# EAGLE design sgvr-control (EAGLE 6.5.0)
CNAME: SGVR Control Board; CREVISION: 1; DESIGNER: Rian Wardana

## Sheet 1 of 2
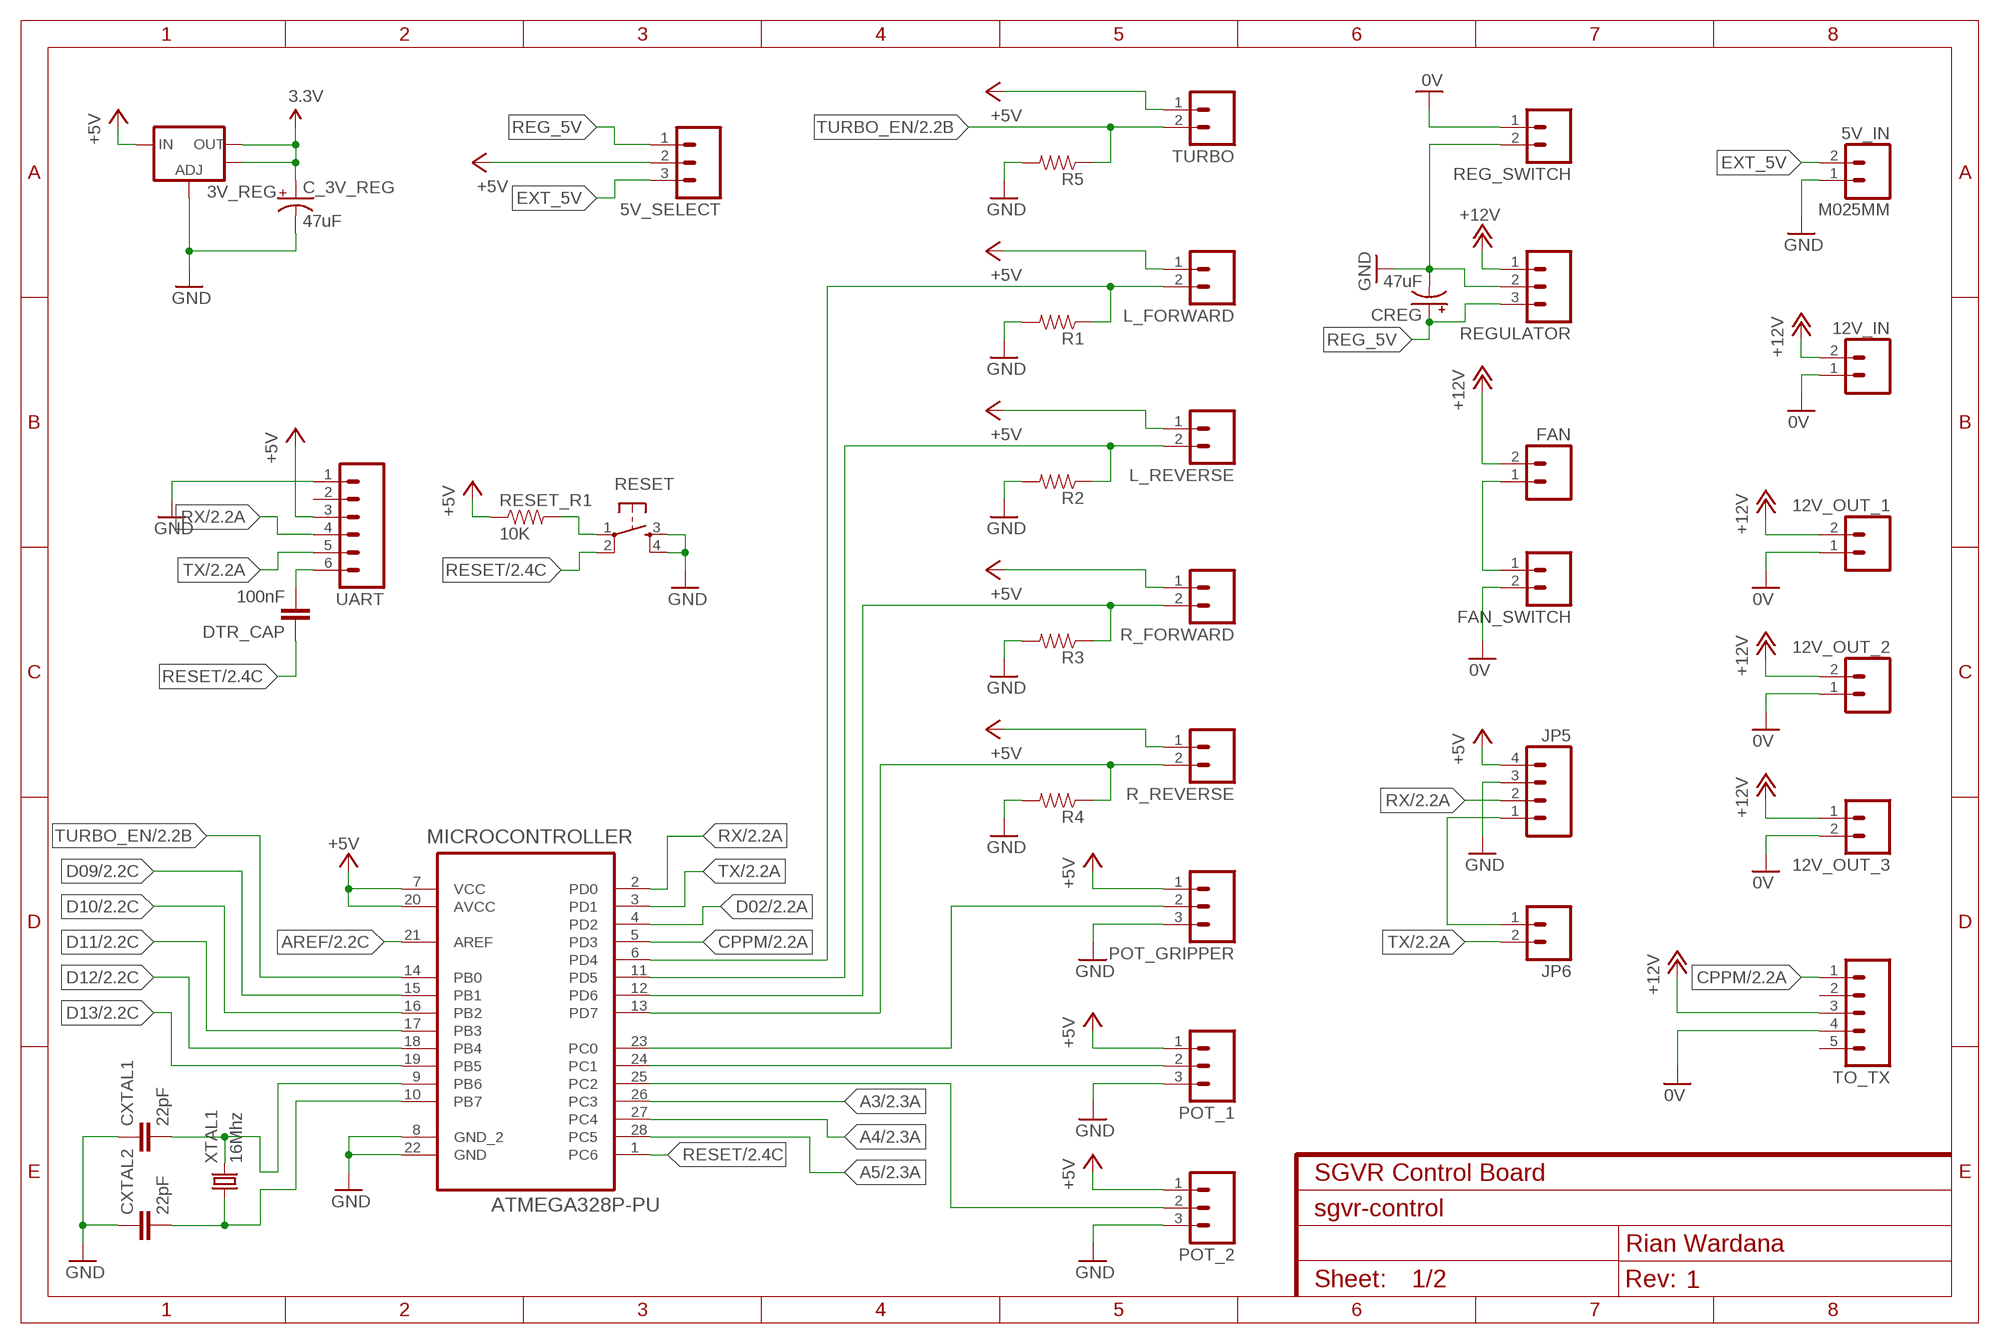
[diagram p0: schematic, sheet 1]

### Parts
3V_REG  V_REG_LM1117SOT223  [SOT223]
5V_IN  M025MM  [SCREWTERMINAL-5MM-2]
5V_SELECT  M03LOCK_LONGPADS  [1X03_LOCK_LONGPADS]
12V_IN  M025MM  [SCREWTERMINAL-5MM-2]
12V_OUT_1  M025MM  [SCREWTERMINAL-5MM-2]
12V_OUT_2  M025MM  [SCREWTERMINAL-5MM-2]
12V_OUT_3  M02LOCK_LONGPADS  [1X02_LOCK_LONGPADS]
C_3V_REG  47uF  CAP_POLPTH1  [CPOL-RADIAL-100UF-25V]
CREG  47uF  CAP_POLPTH1  [CPOL-RADIAL-100UF-25V]
CXTAL1  22pF  CAPPTH  [CAP-PTH-SMALL]
CXTAL2  22pF  CAPPTH  [CAP-PTH-SMALL]
DTR_CAP  100nF  CAPPTH  [CAP-PTH-SMALL]
FAN  M02LOCK_LONGPADS  [1X02_LOCK_LONGPADS]
FAN_SWITCH  M02LOCK_LONGPADS  [1X02_LOCK_LONGPADS]
JP5  M04LOCK_LONGPADS  [1X04_LOCK_LONGPADS]
JP6  M02LOCK_LONGPADS  [1X02_LOCK_LONGPADS]
L_FORWARD  M02LOCK_LONGPADS  [1X02_LOCK_LONGPADS]
L_REVERSE  M02LOCK_LONGPADS  [1X02_LOCK_LONGPADS]
MICROCONTROLLER  ATMEGA328P-PU  [DIP254P762X457-28]
POT_1  M03LOCK_LONGPADS  [1X03_LOCK_LONGPADS]
POT_2  M03LOCK_LONGPADS  [1X03_LOCK_LONGPADS]
POT_GRIPPER  M03LOCK_LONGPADS  [1X03_LOCK_LONGPADS]
R1  RESISTORAXIAL-0.3  [AXIAL-0.3]
R2  RESISTORAXIAL-0.3  [AXIAL-0.3]
R3  RESISTORAXIAL-0.3  [AXIAL-0.3]
R4  RESISTORAXIAL-0.3  [AXIAL-0.3]
R5  RESISTORAXIAL-0.3  [AXIAL-0.3]
R_FORWARD  M02LOCK_LONGPADS  [1X02_LOCK_LONGPADS]
R_REVERSE  M02LOCK_LONGPADS  [1X02_LOCK_LONGPADS]
REG_SWITCH  M02LOCK_LONGPADS  [1X02_LOCK_LONGPADS]
REGULATOR  M03LOCK_LONGPADS  [1X03_LOCK_LONGPADS]
RESET  TAC_SWITCHPTH  [TACTILE-PTH]
RESET_R1  10K  RESISTORAXIAL-0.3  [AXIAL-0.3]
TO_TX  M05LOCK_LONGPADS  [1X05_LOCK_LONGPADS]
TURBO  M02LOCK_LONGPADS  [1X02_LOCK_LONGPADS]
UART  M06LOCK_LONGPADS  [1X06_LOCK_LONGPADS]
XTAL1  16Mhz  CRYSTALHC49UV  [HC49U-V]

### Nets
3.3V: 3V_REG.2(OUT) 3V_REG.4(OUT) C_3V_REG.1(+) ; also sheet 2
+5V: 3V_REG.3(IN) 5V_SELECT.2 JP5.4 L_FORWARD.1 L_REVERSE.1 MICROCONTROLLER.7(VCC) MICROCONTROLLER.20(AVCC) POT_1.1 POT_2.1 POT_GRIPPER.1 R_FORWARD.1 R_REVERSE.1 RESET_R1.P$1 TURBO.1 UART.3 ; also sheet 2
+12V: 12V_IN.2 12V_OUT_1.2 12V_OUT_2.2 12V_OUT_3.1 FAN.2 REGULATOR.1 TO_TX.3
A0: MICROCONTROLLER.23(PC0) POT_GRIPPER.2 ; also sheet 2
A1: MICROCONTROLLER.24(PC1) POT_1.2 ; also sheet 2
A2: MICROCONTROLLER.25(PC2) POT_2.2 ; also sheet 2
A3: MICROCONTROLLER.26(PC3) ; also sheet 2
A4: MICROCONTROLLER.27(PC4) ; also sheet 2
A5: MICROCONTROLLER.28(PC5) ; also sheet 2
AREF: MICROCONTROLLER.21(AREF) ; also sheet 2
CPPM: MICROCONTROLLER.5(PD3) TO_TX.1 ; also sheet 2
D02: MICROCONTROLLER.4(PD2) ; also sheet 2
D04: L_FORWARD.2 MICROCONTROLLER.6(PD4) R1.P$1 ; also sheet 2
D05: L_REVERSE.2 MICROCONTROLLER.11(PD5) R2.P$1 ; also sheet 2
D06: MICROCONTROLLER.12(PD6) R3.P$1 R_FORWARD.2 ; also sheet 2
D07: MICROCONTROLLER.13(PD7) R4.P$1 R_REVERSE.2 ; also sheet 2
D09: MICROCONTROLLER.15(PB1) ; also sheet 2
D10: MICROCONTROLLER.16(PB2) ; also sheet 2
D12: MICROCONTROLLER.18(PB4) ; also sheet 2
D13: MICROCONTROLLER.19(PB5) ; also sheet 2
DTR: DTR_CAP.2 UART.6
EXT_5V: 5V_IN.2 5V_SELECT.3
GND: 3V_REG.1(ADJ) 5V_IN.1 C_3V_REG.2(-) CREG.2(-) CXTAL1.1 CXTAL2.1 JP5.3 MICROCONTROLLER.8(GND_2) MICROCONTROLLER.22(GND) POT_1.3 POT_2.3 POT_GRIPPER.3 R1.P$2 R2.P$2 R3.P$2 R4.P$2 R5.P$2 REG_SWITCH.2 REGULATOR.2 RESET.3 RESET.4 UART.1 ; also sheet 2
GROUND12: 12V_IN.1 12V_OUT_1.1 12V_OUT_2.1 12V_OUT_3.2 FAN_SWITCH.2 REG_SWITCH.1 TO_TX.4 ; supply symbol labelled 0V
N$1: FAN.1 FAN_SWITCH.1
N$2: JP5.1 JP6.1
N$3: CXTAL1.2 MICROCONTROLLER.9(PB6) XTAL1.2
N$4: CXTAL2.2 MICROCONTROLLER.10(PB7) XTAL1.1
N$13: RESET.1 RESET_R1.P$2
REG_5V: 5V_SELECT.1 CREG.1(+) REGULATOR.3
RESET: DTR_CAP.1 MICROCONTROLLER.1(PC6) RESET.2 ; also sheet 2
RX: JP5.2 MICROCONTROLLER.2(PD0) UART.4 ; also sheet 2
TURBO_EN: MICROCONTROLLER.14(PB0) R5.P$1 TURBO.2 ; also sheet 2
TX: JP6.2 MICROCONTROLLER.3(PD1) UART.5 ; also sheet 2
Unconnected: MICROCONTROLLER.17(PB3) TO_TX.2 TO_TX.5 UART.2

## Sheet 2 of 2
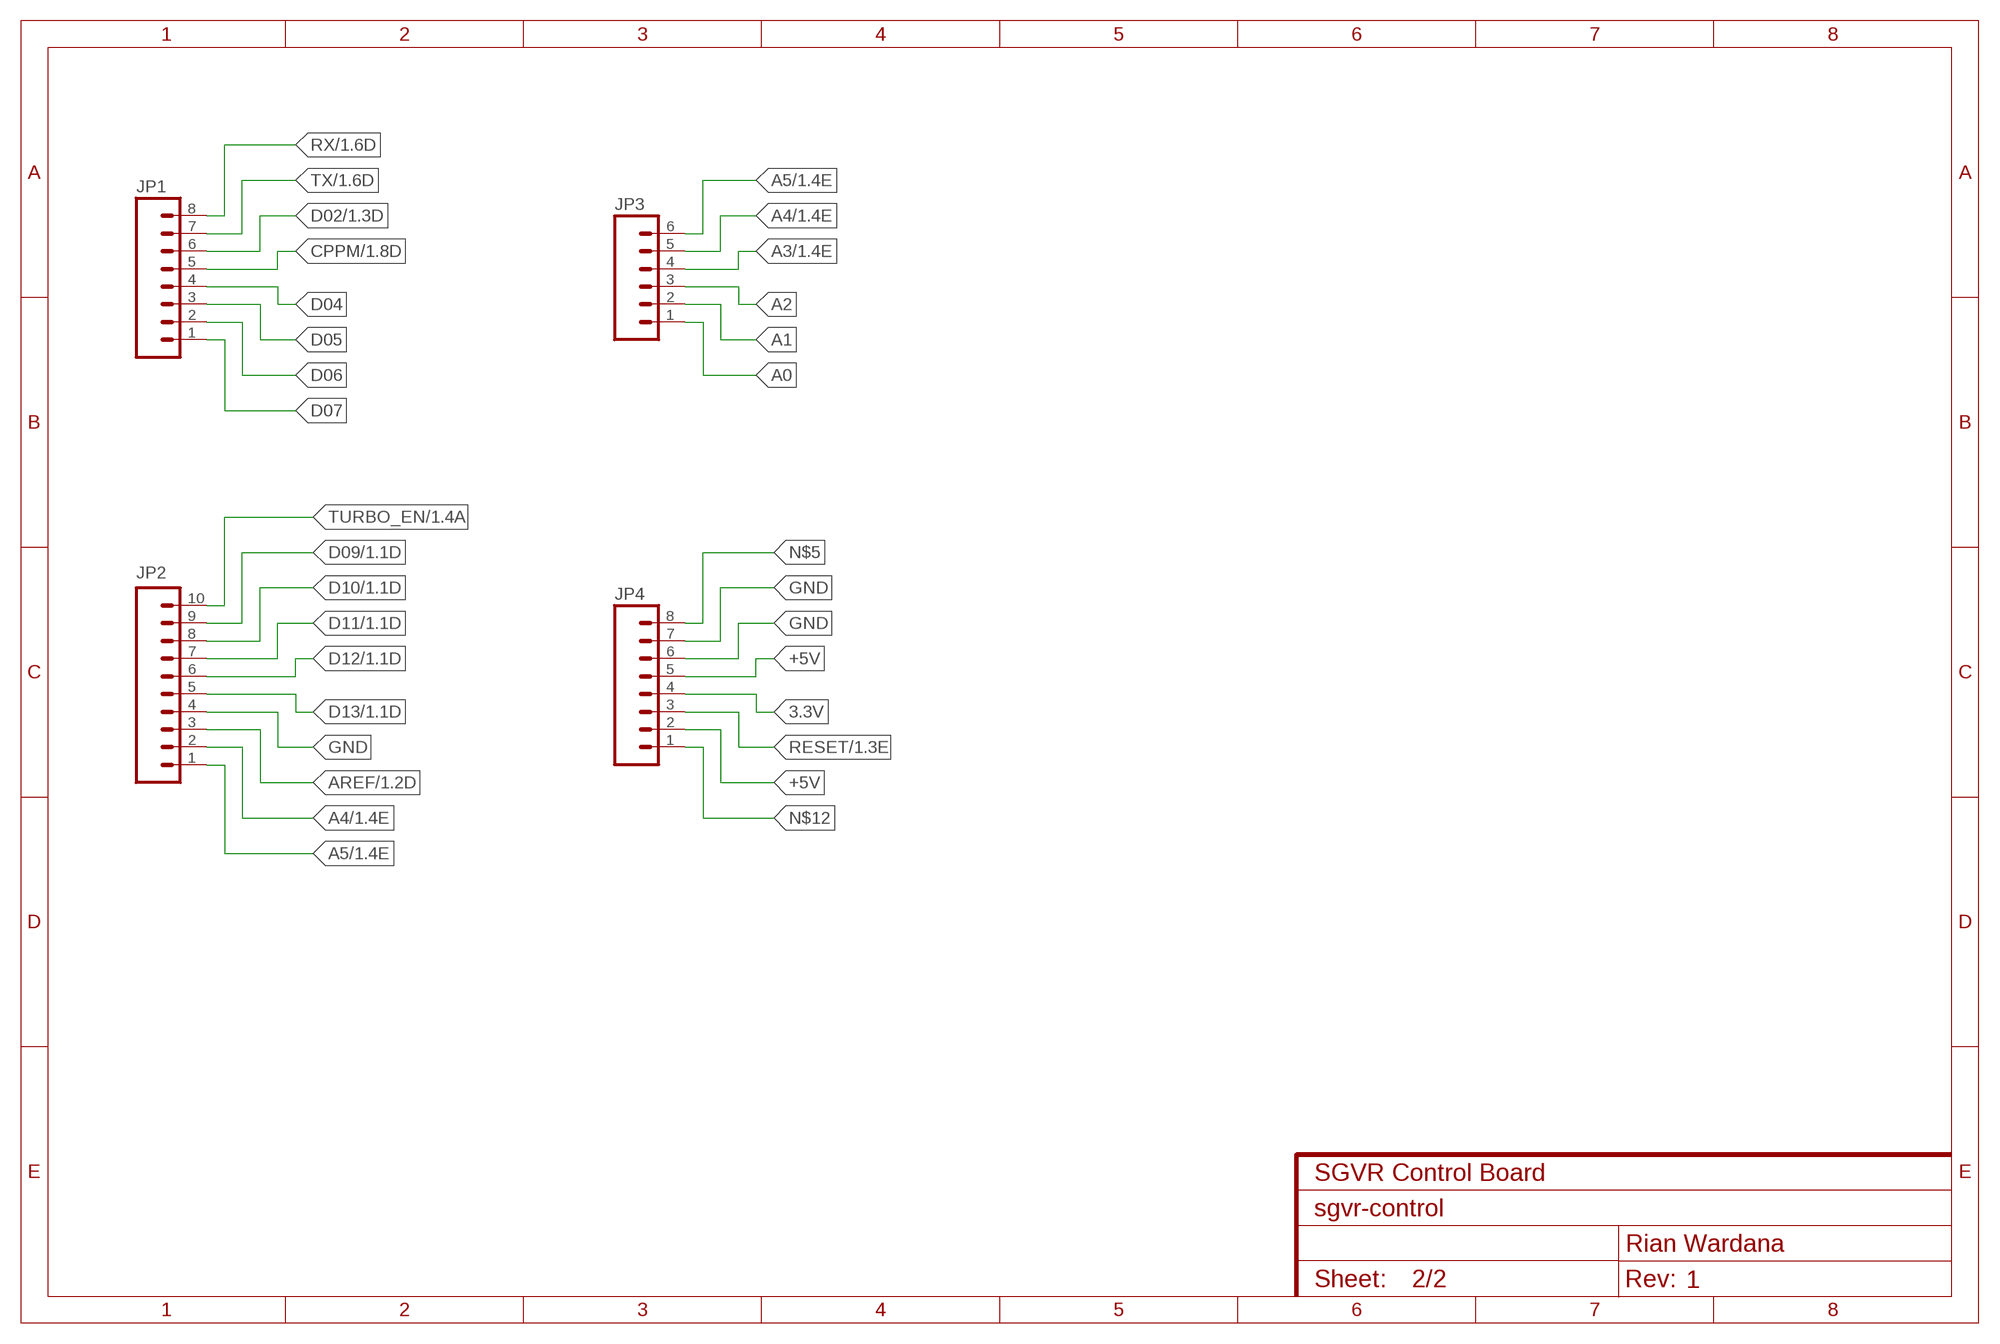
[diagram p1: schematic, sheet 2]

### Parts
JP1  M08LOCK_LONGPADS  [1X08_LOCK_LONGPADS]
JP2  M10LOCK_LONGPADS  [1X10_LOCK_LONGPADS]
JP3  M06LOCK_LONGPADS  [1X06_LOCK_LONGPADS]
JP4  M08LOCK_LONGPADS  [1X08_LOCK_LONGPADS]

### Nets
3.3V: JP4.4 ; also sheet 1
+5V: JP4.2 JP4.5 ; also sheet 1
A0: JP3.1 ; also sheet 1
A1: JP3.2 ; also sheet 1
A2: JP3.3 ; also sheet 1
A3: JP3.4 ; also sheet 1
A4: JP2.2 JP3.5 ; also sheet 1
A5: JP2.1 JP3.6 ; also sheet 1
AREF: JP2.3 ; also sheet 1
CPPM: JP1.5 ; also sheet 1
D02: JP1.6 ; also sheet 1
D04: JP1.4 ; also sheet 1
D05: JP1.3 ; also sheet 1
D06: JP1.2 ; also sheet 1
D07: JP1.1 ; also sheet 1
D09: JP2.9 ; also sheet 1
D10: JP2.8 ; also sheet 1
D11: JP2.7 ; also sheet 1
D12: JP2.6 ; also sheet 1
D13: JP2.5 ; also sheet 1
GND: JP2.4 JP4.6 JP4.7 ; also sheet 1
N$5: JP4.8
N$12: JP4.1
RESET: JP4.3 ; also sheet 1
RX: JP1.8 ; also sheet 1
TURBO_EN: JP2.10 ; also sheet 1
TX: JP1.7 ; also sheet 1

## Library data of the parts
3V_REG = SparkFun-PowerIC:V_REG_LM1117: Voltage Regulator LM1117 Standard adjustable voltage regulator but in SMD form. Spark Fun Electronics SKU : COM-00595
5V_IN 12V_IN 12V_OUT_1-12V_OUT_3 FAN FAN_SWITCH JP6 L_FORWARD L_REVERSE R_FORWARD R_REVERSE REG_SWITCH TURBO = SparkFun-Connectors:M02: Standard 2-pin 0.1" header. Use with
5V_SELECT POT_1 POT_2 POT_GRIPPER REGULATOR = SparkFun-Connectors:M03: Header 3 Standard 3-pin 0.1" header. Use with straight break away headers (SKU : PRT-00116), right angle break away headers (PRT-00553), swiss pins (PRT-00743), machine pins (PRT-00117), and female headers (PRT-00115). Molex polarized connector foot print use with SKU : PRT-08232 with associated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
C_3V_REG = SparkFun-Capacitors:CAP_POL: Capacitor Polarized
CREG = SparkFun-Passives:CAP_POL: Capacitor Polarized
CXTAL1 CXTAL2 DTR_CAP = SparkFun-Capacitors:CAP: Capacitor
JP1 JP4 = SparkFun-Connectors:M08: Header 8 Standard 8-pin 0.1" header. Use with straight break away headers (SKU : PRT-00116), right angle break away headers (PRT-00553), swiss pins (PRT-00743), machine pins (PRT-00117), and female headers (PRT-00115).
JP2 = SparkFun-Connectors:M10: Header 10 Standard 10-pin 0.1" header. Use with straight break away headers (SKU : PRT-00116), right angle break away headers (PRT-00553), swiss pins (PRT-00743), machine pins (PRT-00117), and female headers (PRT-00115).
JP3 UART = SparkFun-Connectors:M06: Header 6 Standard 6-pin 0.1" header. Use with straight break away headers (SKU : PRT-00116), right angle break away headers (PRT-00553), swiss pins (PRT-00743), machine pins (PRT-00117), and female headers (PRT-00115). Molex polarized connector foot print use with SKU : PRT-08094 with associated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
JP5 = SparkFun-Connectors:M04: Header 4 Standard 4-pin 0.1" header. Use with straight break away headers (SKU : PRT-00116), right angle break away headers (PRT-00553), swiss pins (PRT-00743), machine pins (PRT-00117), and female headers (PRT-00115). Molex polarized connector foot print use with SKU : PRT-08231 with associated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
MICROCONTROLLER = Atmel_By_element14_Batch_1-00:ATMEGA328P-PU: 8-bit Microcontroller with In-System Programmable Flash; MPN: ATMEGA328P-PU; OC_FARNELL: 1715487; OC_NEWARK: 15R0268; PACKAGE: PDIP-28; SUPPLIER: Atmel
R1-R5 RESET_R1 = SparkFun-Resistors:RESISTOR: Resistor
RESET = SparkFun-Electromechanical:TAC_SWITCH: Momentary Switch Button commonly used for reset or general input. Spark Fun Electronics SKU : COM-00097 SMT- SWCH-08247
TO_TX = SparkFun-Connectors:M05: Header 5 Standard 5-pin 0.1" header. Use with straight break away headers (SKU : PRT-00116), right angle break away headers (PRT-00553), swiss pins (PRT-00743), machine pins (PRT-00117), and female headers (PRT-00115). Molex polarized connector foot print use with SKU : PRT-08230 with associated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
XTAL1 = SparkFun-FreqCtrl:CRYSTAL: Various standard crystals. Proven footprints. Spark Fun Electronics SKU : COM-00534

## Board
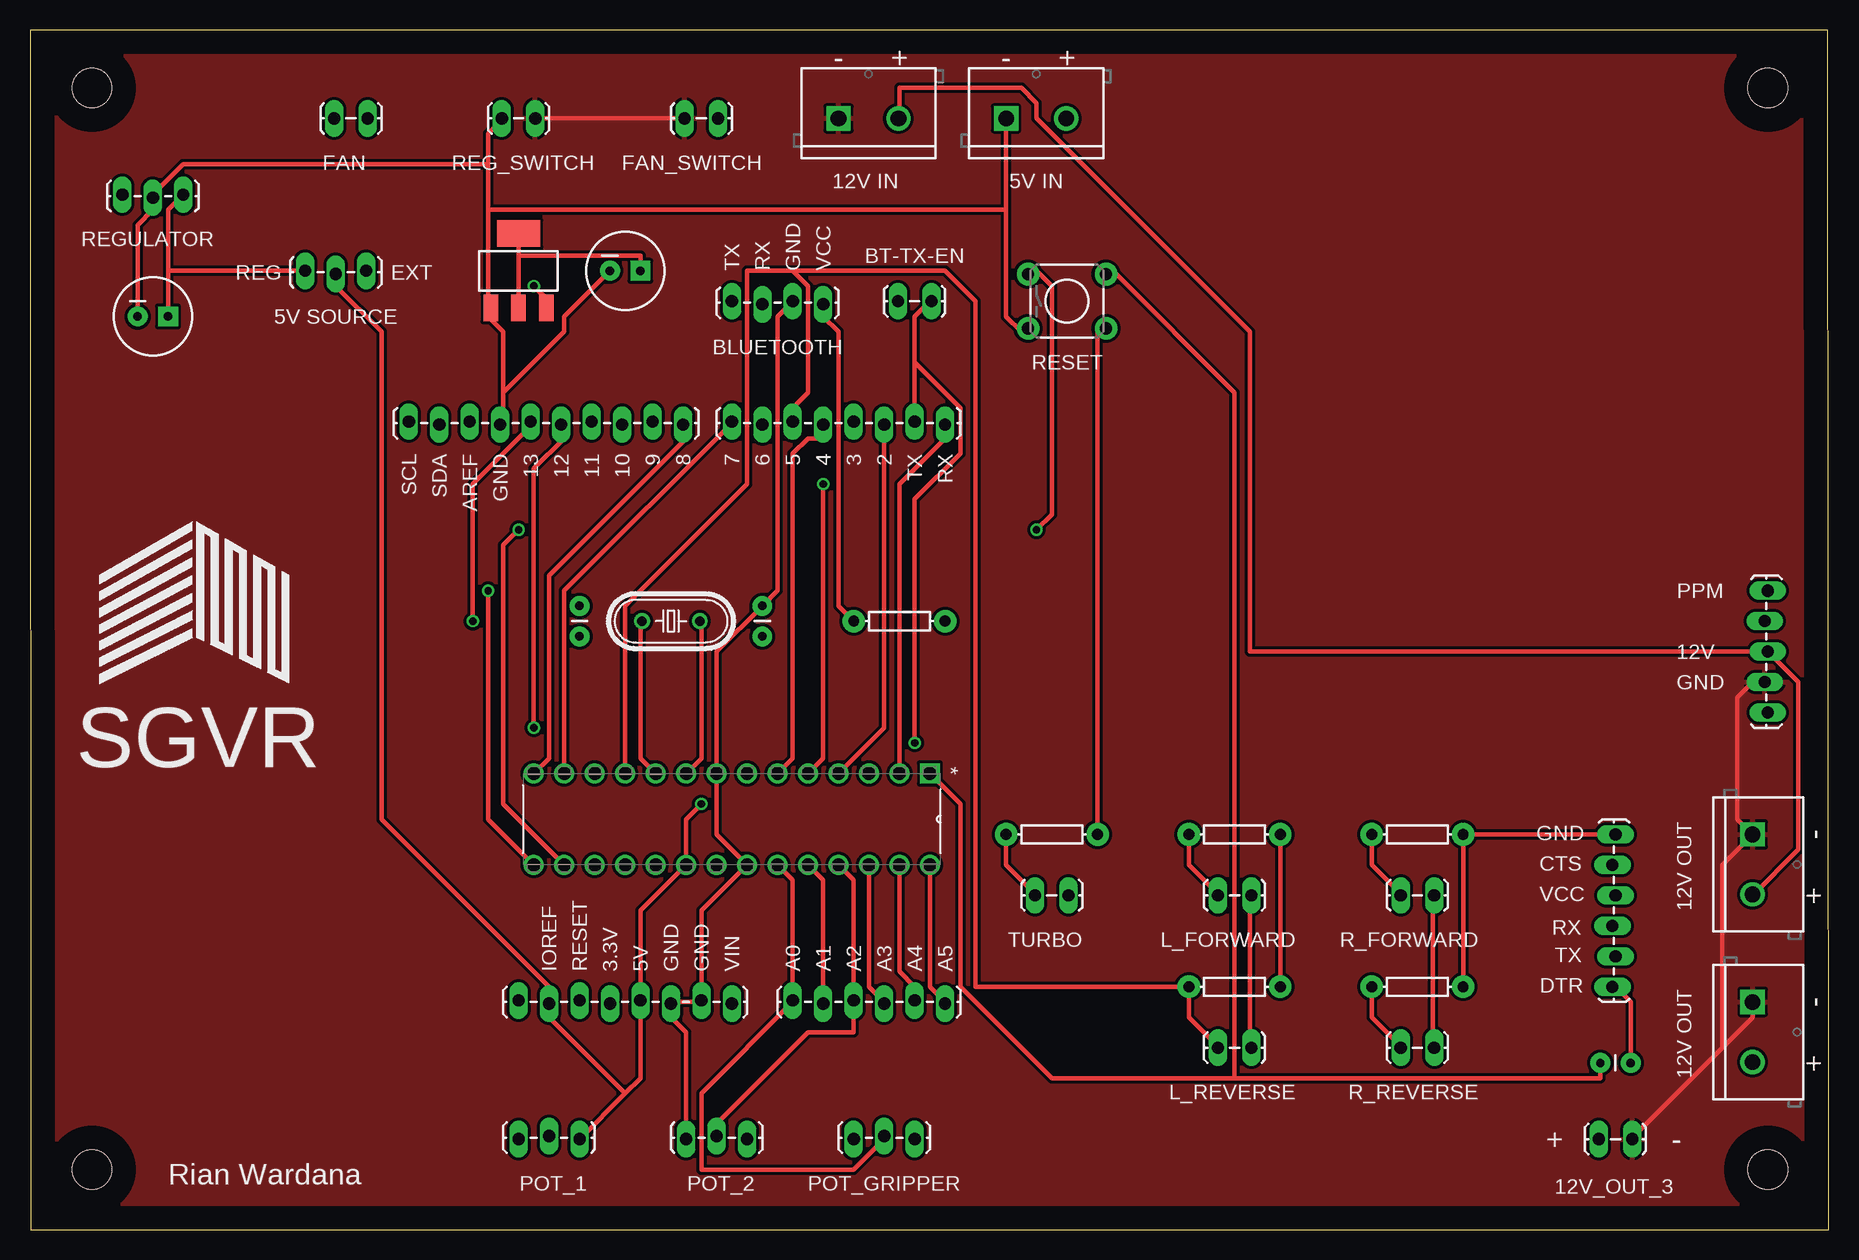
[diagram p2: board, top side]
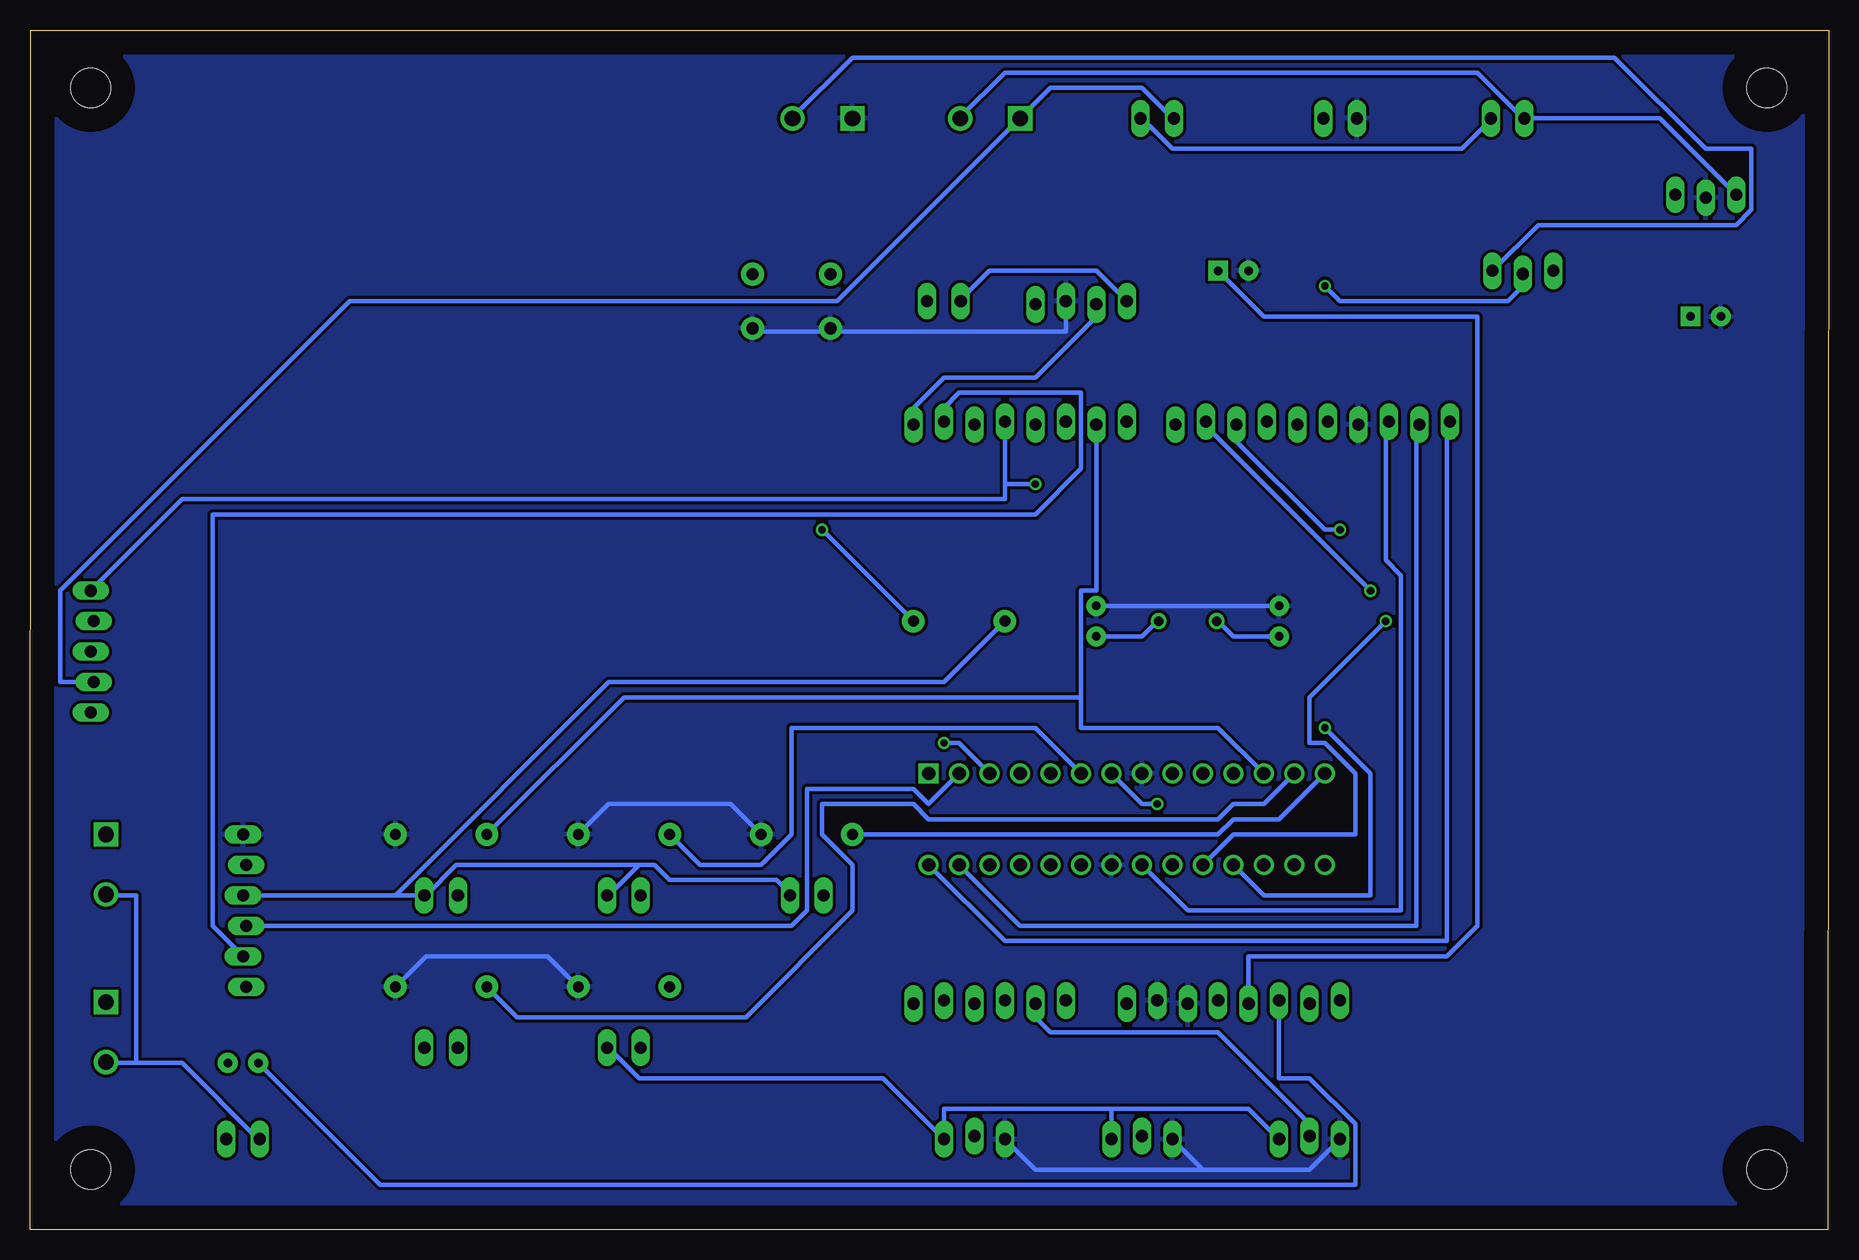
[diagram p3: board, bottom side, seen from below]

Size 149.92 x 100 mm. Coordinates in mm from the lower left corner, seen from the top.
Outline: 0.08,0 149.92,0 149.84,100 0,100 0.08,0
Copper layers (1*16): Top 0.035mm / dielectric 1.5mm / Bottom 0.035mm
Design rules "Mazmood *": minimum track width 15mil, minimum drill 24mil, track to track 10mil, track to pad 10mil, pad to pad 10mil, via to via 10mil, smd to smd 10mil, copper to edge 2mm, drill to drill 10mil, minimum pad ring 10mil, minimum via ring 8mil, stop-mask expansion 4mil, vias tented up to drill 0mil, thermal gap 10mil

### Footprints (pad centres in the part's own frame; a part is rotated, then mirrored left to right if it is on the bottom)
SOT223 = smd 1.219 x 2.235: 1 -2.311,-3.099; 2 0,-3.099; 3 2.311,-3.099 | smd 3.6 x 2.2: 4 0,3.099
SCREWTERMINAL-5MM-2 = drill 1.3 pad 2.032 square: 1 0,0 | drill 1.3 pad 2.032: 2 5,0
1X03_LOCK_LONGPADS = drill 1.016 long: 1 0,0; 2 2.54,-0.254; 3 5.08,0
1X02_LOCK_LONGPADS = drill 1.016 long: 1 -0.127,0; 2 2.667,0
CPOL-RADIAL-100UF-25V = drill 0.7 pad 1.651 square: 1 1.27,0 | drill 0.7 pad 1.651: 2 -1.27,0
CAP-PTH-SMALL = drill 0.7 pad 1.651: 1 0,0; 2 2.54,0
1X08_LOCK_LONGPADS = drill 1.016 long: 1 0,0.127; 2 2.54,-0.127; 3 5.08,0.127; 4 7.62,-0.127; 5 10.16,0.127; 6 12.7,-0.127; 7 15.24,0.127; 8 17.78,-0.127
1X10_LOCK_LONGPADS = drill 1.016 long: 1 0,0.127; 2 2.54,-0.127; 3 5.08,0.127; 4 7.62,-0.127; 5 10.16,0.127; 6 12.7,-0.127; 7 15.24,0.127; 8 17.78,-0.127; 9 20.32,0.127; 10 22.86,-0.127
1X06_LOCK_LONGPADS = drill 1.016 long: 1 0,0; 2 2.54,-0.254; 3 5.08,0; 4 7.62,-0.254; 5 10.16,0; 6 12.7,-0.254
1X04_LOCK_LONGPADS = drill 1.016 long: 1 0,0; 2 2.54,-0.254; 3 5.08,0; 4 7.62,-0.254
DIP254P762X457-28 = drill 1.118 square: 1 -7.62,33.02 | drill 1.118: 2 -7.62,30.48; 3 -7.62,27.94; 4 -7.62,25.4; 5 -7.62,22.86; 6 -7.62,20.32; 7 -7.62,17.78; 8 -7.62,15.24; 9 -7.62,12.7; 10 -7.62,10.16; 11 -7.62,7.62; 12 -7.62,5.08; 13 -7.62,2.54; 14 -7.62,0; 15 0,0; 16 0,2.54; 17 0,5.08; 18 0,7.62; 19 0,10.16; 20 0,12.7; 21 0,15.24; 22 0,17.78; 23 0,20.32; 24 0,22.86; 25 0,25.4; 26 0,27.94; 27 0,30.48; 28 0,33.02
AXIAL-0.3 = drill 0.9 pad 1.88: P$1 -3.81,0; P$2 3.81,0
TACTILE-PTH = drill 1.016 pad 1.88: 1 -3.251,2.261; 2 3.251,2.261; 3 -3.251,-2.261; 4 3.251,-2.261
1X05_LOCK_LONGPADS = drill 1.016 long: 1 0,0; 2 2.54,-0.254; 3 5.08,0; 4 7.62,-0.254; 5 10.16,0
STAND-OFF = hole 3.302: 0,0
HC49U-V = drill 0.813: 1 -2.413,0; 2 2.413,0

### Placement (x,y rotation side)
3V_REG  40.72,79.93 0 top
5V_IN  81.36,92.63 0 top
5V_SELECT  22.94,79.93 0 top
12V_IN  67.39,92.63 0 top
12V_OUT_1  143.59,32.94 270 top
12V_OUT_2  143.59,18.97 270 top
12V_OUT_3  130.89,7.54 0 top
C_3V_REG  49.61,79.93 0 top
CREG  10.24,76.12 0 top
CXTAL1  61.04,51.99 270 top
CXTAL2  45.8,51.99 270 top
DTR_CAP  130.89,13.89 0 top
FAN  28.02,92.63 180 top
FAN_SWITCH  57.23,92.63 180 top
JP1  58.5,67.23 0 top
JP2  31.58,67.23 0 top
JP3  63.58,19.1 0 top
JP4  40.72,18.97 0 top
JP5  58.5,77.39 0 top
JP6  72.47,77.39 0 top
L_FORWARD  101.68,27.86 180 top
L_REVERSE  101.68,15.16 180 top
MICROCONTROLLER  41.99,30.4 270 top
POT_1  45.8,7.54 180 top
POT_2  59.77,7.54 180 top
POT_GRIPPER  73.74,7.54 180 top
R1  100.41,32.94 0 top
R2  100.41,20.24 0 top
R3  115.65,32.94 0 top
R4  115.65,20.24 0 top
R5  85.17,32.94 0 top
R_FORWARD  116.92,27.86 180 top
R_REVERSE  116.92,15.16 180 top
REG_SWITCH  41.99,92.63 180 top
REGULATOR  7.7,86.28 0 top
RESET  86.44,77.39 0 top
RESET_R1  72.47,50.72 0 top
TO_TX  144.86,53.26 270 top
TURBO  86.44,27.86 180 top
U$1  [STAND-OFF]  144.86,5 0 top
U$2  [STAND-OFF]  5.16,5 0 top
U$3  [STAND-OFF]  5.16,95.17 0 top
U$4  [STAND-OFF]  144.86,95.17 0 top
UART  132.16,32.94 270 top
XTAL1  53.42,50.72 0 top

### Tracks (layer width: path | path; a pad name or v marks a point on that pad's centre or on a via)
3.3V
  Top 0.381: 3V_REG.4 40.72,81.2 | 40.72,81.2 3V_REG.2 | 40.72,81.2 50.88,81.2 C_3V_REG.1
  Bottom 0.381: JP4.4 48.34,22.78 31.83,22.78 29.29,25.32 29.29,76.12 47.07,76.12 C_3V_REG.1
+5V  (via drill 0.61)
  Top 0.381: v41.99,78.66 43.26,77.39 3V_REG.3 | 49.61,11.35 50.88,12.62 JP4.5 50.88,26.59 MICROCONTROLLER.20 54.69,34.21 v55.96,35.48 | 49.61,11.35 POT_1.1 | 49.61,11.35 43.26,17.7 JP4.2 43.26,20.24 29.29,34.21 29.29,74.85 25.48,78.66 5V_SELECT.2 | RESET_R1.P$1 67.39,51.99 67.39,74.85 66.12,76.12 JP5.4 | R_REVERSE.1 116.92,15.16 116.92,27.86 R_FORWARD.1 | L_REVERSE.1 101.68,15.16 101.68,27.86 L_FORWARD.1
  Bottom 0.381: v41.99,78.66 40.72,77.39 26.75,77.39 25.48,78.66 5V_SELECT.2 | 59.77,10.08 POT_2.1 | 59.77,10.08 48.34,10.08 POT_1.1 | 59.77,10.08 73.74,10.08 POT_GRIPPER.1 78.82,12.62 99.14,12.62 101.68,15.16 L_REVERSE.1 | MICROCONTROLLER.7 57.23,35.48 v55.96,35.48 | 119.46,27.86 R_FORWARD.1 116.92,27.86 114.38,30.4 99.14,30.4 | 119.46,27.86 UART.3 | 99.14,30.4 97.87,30.4 96.6,29.13 87.71,29.13 86.44,27.86 TURBO.1 | 99.14,30.4 101.68,27.86 L_FORWARD.1 | RESET_R1.P$1 73.74,45.64 101.68,45.64 119.46,27.86
+12V
  Top 0.381: 12V_OUT_1.2 143.59,27.86 147.4,31.67 147.4,45.64 TO_TX.3 101.68,48.18 101.68,74.85 83.9,92.63 83.9,93.9 82.63,95.17 72.47,95.17 72.47,92.63 12V_IN.2
  Bottom 0.381: 141.05,13.89 143.59,13.89 12V_OUT_2.2 | 141.05,13.89 137.24,13.89 130.89,7.54 12V_OUT_3.1 | 141.05,13.89 141.05,27.86 143.59,27.86 12V_OUT_1.2 | REGULATOR.1 14.05,92.63 FAN.2 25.48,92.63 29.29,96.44 68.66,96.44 72.47,92.63 12V_IN.2
A0
  Top 0.381: POT_GRIPPER.2 71.2,7.54 68.66,5 55.96,5 55.96,11.35 63.58,18.97 JP3.1 63.58,29.13 MICROCONTROLLER.23
A1
  Top 0.381: MICROCONTROLLER.24 66.12,29.13 JP3.2
  Bottom 0.381: POT_1.2 43.26,8.81 50.88,16.43 64.85,16.43 66.12,17.7 JP3.2
A2
  Top 0.381: POT_2.2 57.23,8.81 64.85,16.43 68.66,16.43 JP3.3 68.66,29.13 MICROCONTROLLER.25
A3
  Top 0.381: MICROCONTROLLER.26 69.93,20.24 71.2,18.97 JP3.4
A4
  Top 0.381: MICROCONTROLLER.27 72.47,21.51 73.74,20.24 JP3.5
  Bottom 0.381: MICROCONTROLLER.27 67.39,25.32 34.37,25.32 34.37,65.96 JP2.2
A5
  Top 0.381: MICROCONTROLLER.28 75.01,20.24 76.28,18.97 JP3.6
  Bottom 0.381: MICROCONTROLLER.28 68.66,24.05 31.83,24.05 31.83,67.23 JP2.1
AREF
  Bottom 0.381: MICROCONTROLLER.21 53.42,26.59 35.64,26.59 35.64,54.53 36.91,55.8 36.91,67.23 JP2.3
CPPM  (via drill 0.61)
  Top 0.381: MICROCONTROLLER.5 66.12,39.29 v66.12,62.15
  Bottom 0.381: 68.66,62.15 68.66,60.88 137.24,60.88 TO_TX.1 | 68.66,62.15 JP1.5 | 68.66,62.15 v66.12,62.15
D02
  Top 0.381: JP1.6 71.2,41.83 MICROCONTROLLER.4
D04
  Top 0.381: R1.P$1 96.6,30.4 99.14,27.86 L_FORWARD.2 | MICROCONTROLLER.6 63.58,39.29 63.58,64.69 64.85,65.96 66.12,65.96 JP1.4
  Bottom 0.381: R1.P$1 94.06,30.4 88.98,30.4 86.44,32.94 86.44,41.83 66.12,41.83 MICROCONTROLLER.6
D05
  Top 0.381: L_REVERSE.2 99.14,15.16 96.6,17.7 R2.P$1 78.82,20.24 78.82,77.39 76.28,79.93 63.58,79.93 | 63.58,79.93 64.85,78.66 64.85,69.77 63.58,68.5 JP1.3 | 63.58,79.93 59.77,79.93 59.77,62.15 49.61,51.99 MICROCONTROLLER.11
D06
  Top 0.381: R3.P$1 111.84,30.4 114.38,27.86 R_FORWARD.2
  Bottom 0.381: JP1.2 61.04,53.26 62.31,53.26 62.31,44.37 | 62.31,44.37 62.31,41.83 50.88,41.83 MICROCONTROLLER.12 | R3.P$1 100.41,44.37 62.31,44.37
D07
  Top 0.381: R4.P$1 111.84,17.7 114.38,15.16 R_REVERSE.2 | MICROCONTROLLER.13 44.53,53.26 58.5,67.23 JP1.1
  Bottom 0.381: R4.P$1 109.3,17.7 90.25,17.7 81.36,26.59 81.36,30.4 83.9,32.94 83.9,35.48 76.28,35.48 75.01,34.21 50.88,34.21 49.61,35.48 47.07,35.48 MICROCONTROLLER.13
D09  (via drill 0.61)
  Top 0.381: v38.18,53.26 38.18,34.21 MICROCONTROLLER.15
  Bottom 0.381: v38.18,53.26 52.15,67.23 JP2.9
D10  (via drill 0.61)
  Top 0.381: v40.72,58.34 39.45,57.07 39.45,35.48 MICROCONTROLLER.16
  Bottom 0.381: v40.72,58.34 41.99,58.34 49.61,65.96 JP2.8
D12  (via drill 0.61)
  Top 0.381: v41.99,41.83 41.99,63.42 44.53,65.96 JP2.6
  Bottom 0.381: v41.99,41.83 38.18,38.02 38.18,27.86 47.07,27.86 MICROCONTROLLER.18
D13  (via drill 0.61)
  Top 0.381: v36.91,50.72 36.91,62.15 41.99,67.23 JP2.5
  Bottom 0.381: v36.91,50.72 43.26,44.37 43.26,40.56 41.99,40.56 39.45,38.02 39.45,32.94 49.61,32.94 MICROCONTROLLER.19
DTR
  Top 0.381: DTR_CAP.2 133.43,18.97 132.16,20.24 UART.6
EXT_5V
  Bottom 0.381: 5V_SELECT.3 24.21,83.74 7.7,83.74 6.43,85.01 6.43,90.09 10.24,90.09 17.86,97.71 81.36,97.71 86.44,92.63 5V_IN.2
GND
  Top 0.381: POT_2.3 54.69,16.43 53.42,17.7 JP4.6 53.42,18.97 55.96,18.97 JP4.7 55.96,26.59 MICROCONTROLLER.22 57.23,32.94 MICROCONTROLLER.8 57.23,48.18 CXTAL1.1 62.31,53.26 62.31,76.12 JP5.3 | CREG.2 8.97,83.74 10.24,85.01 REGULATOR.2 10.24,86.28 12.78,88.82 38.18,88.82 | 39.45,69.77 39.45,67.23 JP2.4 | 39.45,69.77 39.45,74.85 38.18,76.12 3V_REG.1 38.18,77.39 38.18,85.01 | 38.18,85.01 38.18,88.82 | 38.18,88.82 38.18,91.36 39.45,92.63 REG_SWITCH.2 | C_3V_REG.2 44.53,76.12 44.53,74.85 39.45,69.77 | 81.36,85.01 81.36,76.12 82.63,74.85 RESET.3 | 81.36,85.01 5V_IN.1 | UART.1 R3.P$2 R4.P$2 | R1.P$2 R2.P$2 | R5.P$2 88.98,74.85 RESET.4 | 81.36,85.01 38.18,85.01
  Bottom 0.381: CXTAL1.1 CXTAL2.1 | POT_1.3 43.26,5 52.15,5 | POT_2.3 52.15,5 | POT_GRIPPER.3 66.12,5 52.15,5 | JP5.3 63.58,74.85 82.63,74.85 RESET.3 83.9,74.85 88.98,74.85 RESET.4 | R5.P$2 91.52,35.48 101.68,35.48 R1.P$2 | R4.P$2 116.92,22.78 106.76,22.78 R2.P$2
  pour Bottom: -1.19,101.52 -1.19,-1.35 151.21,-1.35 151.21,101.52
GROUND12
  Top 0.381: 41.99,92.63 REG_SWITCH.1 FAN_SWITCH.2 54.69,92.63 | TO_TX.4 143.59,45.64 142.32,44.37 142.32,34.21 12V_OUT_1.1 141.05,30.4 141.05,15.16 | 141.05,15.16 143.59,17.7 12V_OUT_2.1 | 141.05,15.16 133.43,7.54 12V_OUT_3.2
  Bottom 0.381: FAN_SWITCH.2 54.69,92.63 57.23,95.17 64.85,95.17 12V_IN.1 82.63,77.39 123.27,77.39 147.4,53.26 147.4,45.64 TO_TX.4
  pour Top: -2.46,-2.62 -2.46,102.79 152.48,102.79 152.48,-2.62
N$1
  Bottom 0.381: FAN.1 28.02,92.63 30.56,90.09 54.69,90.09 57.23,92.63 FAN_SWITCH.1
N$2
  Bottom 0.381: JP5.1 61.04,79.93 69.93,79.93 72.47,77.39 JP6.1
N$3
  Top 0.381: MICROCONTROLLER.9 55.96,39.29 55.96,50.72 XTAL1.2
  Bottom 0.381: CXTAL1.2 57.23,49.45 55.96,50.72 XTAL1.2
N$4
  Top 0.381: MICROCONTROLLER.10 50.88,39.29 50.88,50.72 XTAL1.1
  Bottom 0.381: CXTAL2.2 49.61,49.45 50.88,50.72 XTAL1.1
N$13  (via drill 0.61)
  Top 0.381: v83.9,58.34 85.17,59.61 85.17,78.66 83.9,79.93 RESET.1
  Bottom 0.381: v83.9,58.34 RESET_R1.P$2
REG_5V
  Top 0.381: REGULATOR.3 11.51,85.01 11.51,79.93 | CREG.1 11.51,79.93 | 11.51,79.93 5V_SELECT.1
RESET
  Top 0.381: MICROCONTROLLER.1 77.55,35.48 77.55,20.24 85.17,12.62 100.41,12.62 | 100.41,12.62 130.89,12.62 DTR_CAP.1 | 100.41,12.62 100.41,69.77 90.25,79.93 RESET.2
  Bottom 0.381: JP4.3 45.8,12.62 43.26,12.62 39.45,8.81 39.45,3.73 120.73,3.73 DTR_CAP.1
RX
  Top 0.381: MICROCONTROLLER.2 72.47,62.15 76.28,65.96 JP1.8
  Bottom 0.381: UART.4 86.44,25.32 85.17,26.59 85.17,36.75 76.28,36.75 75.01,35.48 MICROCONTROLLER.2 | JP1.8 76.28,68.5 73.74,71.04 66.12,71.04 61.04,76.12 JP5.2
TURBO_EN
  Top 0.381: R5.P$1 81.36,30.4 83.9,27.86 TURBO.2 | MICROCONTROLLER.14 43.26,39.29 43.26,54.53 54.69,65.96 JP2.10
  Bottom 0.381: R5.P$1 50.88,32.94 49.61,34.21 45.8,34.21 MICROCONTROLLER.14
TX  (via drill 0.61)
  Top 0.381: JP1.7 73.74,72.31 | 73.74,72.31 73.74,76.12 75.01,77.39 JP6.2 | v73.74,40.56 73.74,60.88 77.55,64.69 77.55,68.5 73.74,72.31
  Bottom 0.381: UART.5 134.7,25.32 134.7,59.61 66.12,59.61 62.31,63.42 62.31,69.77 72.47,69.77 73.74,68.5 JP1.7 | MICROCONTROLLER.3 72.47,40.56 v73.74,40.56

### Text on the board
tPlace: C:/Users/Chewing Gum/Desktop/logo.bmp
tNames: - | + | - | + | BT-TX-EN | TX | RX | GND | VCC | 5V SOURCE | BLUETOOTH | RESET | SCL | SDA | AREF | GND | 13 | 12 | 11 | 10 | 9 | 8 | 7 | 6 | 5 | 4 | 3 | 2 | TX | RX | - | + | IOREF | RESET | 3.3V | 5V | GND | GND | VIN | A0 | A1 | A2 | A3 | A4 | A5 | - | + | + | -
tSilk: 12V IN | 5V IN | REG | EXT | PPM | 12V | GND | SGVR | GND | CTS | VCC | 12V OUT | RX | TX | DTR | 12V OUT | Rian Wardana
